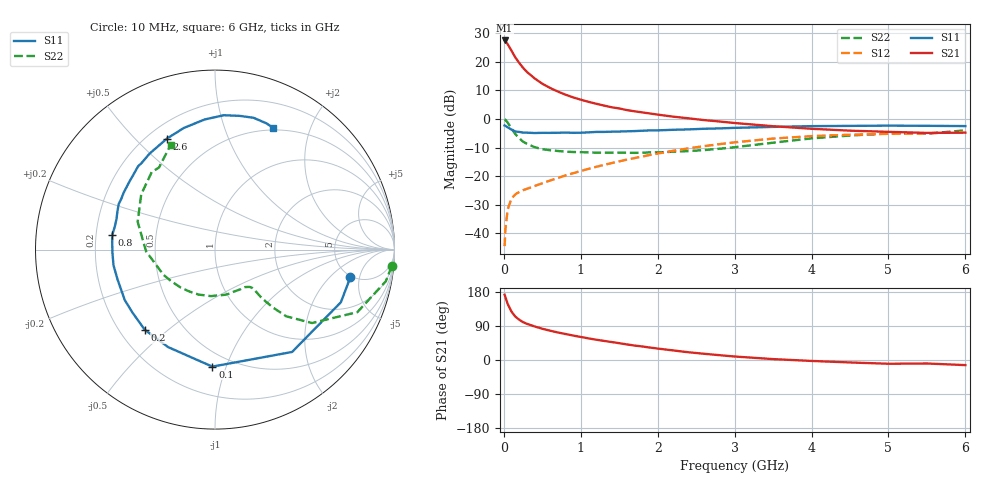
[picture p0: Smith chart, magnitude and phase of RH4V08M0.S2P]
! SIEMENS Small Signal Semiconductors
! BFR106
! Si NPN RF Bipolar Junction Transistor in SOT23
! VCE = 4 V  IC = 8 mA
! Common Emitter S-Parameters:  August  1996
# GHz  S  MA  R  50
!  f  S11  S21  S12  S22
! GHz  MAG  ANG  MAG  ANG  MAG  ANG  MAG  ANG
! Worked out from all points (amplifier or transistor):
!   36 points, 10 MHz to 6 GHz, reference 50 ohm
!   highest |S21| = 27.5 dB at 10 MHz (marker M1)
!   |S21| within 3 dB of that: start of sweep to 86.7 MHz
!   unconditionally stable (mu >= 1): 536.1 MHz to 2.018 GHz; 5.111 GHz to end of sweep
!   at 250 MHz: K = 0.64, MSG = 21.5 dB, |S12| = -25.0 dB
!   at 1.4 GHz: K = 1.11, MAG = 7.8 dB, |S12| = -15.5 dB
!   at 6 GHz: K = 1.02, MAG = -0.9 dB, |S12| = -4.6 dB
!   S11 on the Smith chart (normalised r, x): 10 MHz: 4.82, -3.66; 100 MHz: 0.40, -0.90; 200 MHz: 0.30, -0.42; 800 MHz: 0.27, +0.07; 2.6 GHz: 0.27, +0.62; 6 GHz: 0.47, +1.48
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0.01  0.7697 -11.6  23.83 172.3  0.0059 88.7  0.9885 -5.4
0.02  0.7602 -22.7  23.19 166.2  0.0116 79.8  0.9681 -10.5
0.05  0.714 -53.0  20.49 147.9  0.026 65.9  0.8665 -23.7
0.1  0.6521 -91.3  15.72 127.6  0.0405 51.8  0.6783 -37.1
0.15  0.6028 -115.6  11.98 114.3  0.0478 45.7  0.5443 -43.1
0.2  0.5939 -131.2  9.622 106.3  0.0526 44.0  0.4604 -44.9
0.25  0.5784 -142.7  7.896 99.9  0.0565 44.2  0.4005 -45.7
0.3  0.576 -150.8  6.696 95.5  0.0597 44.9  0.3668 -46.0
0.4  0.5679 -162.8  5.153 88.5  0.0669 47.8  0.3211 -45.7
0.5  0.5722 -171.2  4.161 82.5  0.0747 50.8  0.2959 -45.9
0.6  0.5717 -178.1  3.508 77.4  0.0833 53.7  0.2837 -47.1
0.8  0.5783 171.8  2.674 68.6  0.1022 57.4  0.2678 -51.3
0.9  0.5728 167.3  2.397 64.6  0.1121 58.8  0.264 -53.5
1.1  0.5839 158.6  2.002 57.1  0.1335 60.6  0.2597 -60.5
1.3  0.5938 151.6  1.722 50.5  0.1568 61.3  0.2564 -67.7
1.6  0.6089 141.6  1.434 41.1  0.1939 60.8  0.257 -80.5
2.2  0.647 124.4  1.1 25.3  0.2769 55.9  0.2667 -109.9
2.6  0.6743 113.4  0.958 16.5  0.3338 50.5  0.2849 -132.2
3.5  0.7274 94.5  0.748 2.4  0.4537 35.5  0.3843 -178.6
4.5  0.7576 79.6  0.625 -6.5  0.5302 17.5  0.5135 143.2
5.5  0.7596 67.9  0.571 -9.2  0.5612 5.8  0.5535 124.3
6  0.7519 64.4  0.577 -13.5  0.5906 -2.0  0.6332 113.0
